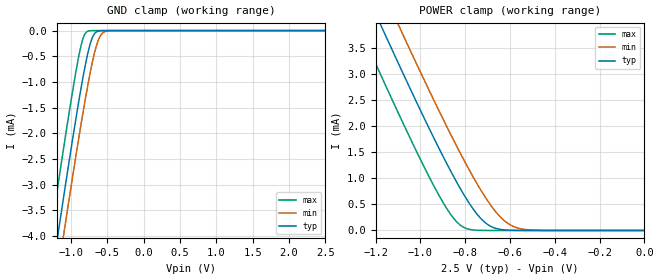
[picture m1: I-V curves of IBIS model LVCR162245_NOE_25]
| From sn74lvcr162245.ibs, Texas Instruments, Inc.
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[Model]   LVCR162245_NOE_25
Model_type  Input
Vinl=0.8
Vinh=2.0
| variable   typ   min   max
C_comp   1.20pF   1.07pF   1.62pF
[Temperature Range]   40   100   -40
| Ambient temperature   25   85   -40
[Voltage range]   2.5   2.3   2.7
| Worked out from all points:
|   GND clamp passes 1 mA (typ) near -0.85 V on its own axis
|   POWER clamp passes 1 mA (typ) near -0.85 V on its own axis
[GND Clamp]
| LVCR162245_NOE_25
|   Voltage   I(typ)   I(min)   I(max)
-5.5V     -46.83mA   -47.49mA   -46mA
-1.28V    -4.92mA    -5.658mA   -3.966mA
-1.18V    -3.971mA   -4.711mA   -3.015mA
-1.1V     -3.223mA   -3.962mA   -2.267mA
-1.075V   -2.991mA   -3.73mA    -2.037mA
-930mV    -1.689mA   -2.412mA   -776uA
-835mV    -905.1uA   -1.593mA   -153.9uA
-765mV    -416uA     -1.031mA   -10.23uA
-705mV    -131.6uA   -603.9uA   -580.2nA
-630mV    -13.33uA   -205.5uA   -15.19nA
-555mV    -923.2nA   -35.19uA   -403.1pA
2.5V      4.712pA    817.5pA    4.189pA
[POWER Clamp]
| LVCR162245_NOE_25
|   Voltage   I(typ)   I(min)   I(max)
-5.5V     46.83mA    47.49mA    46mA
-1.325V   5.35mA     6.087mA    4.398mA
-1.26V    4.729mA    5.468mA    3.775mA
-1.155V   3.736mA    4.476mA    2.78mA
-1.085V   3.084mA    3.822mA    2.129mA
-935mV    1.732mA    2.457mA    816uA
-840mV    943.8uA    1.634mA    176.2uA
-795mV    611.2uA    1.266mA    38.41uA
-725mV    207uA      738.7uA    1.527uA
-620mV    9.413uA    169.2uA    9.344nA
-500mV    126.5nA    7.204uA    33.97pA
-95.1fV   4.712pA    6.41pA     4.886pA
